FUNCTION "SINCRONIZZAZIONE ASSI" : VOID
TITLE =CICLO DI SINCRONIZZAZIONE ASSI
VERSION : 0.1

BEGIN
NETWORK
TITLE =INIZIO SINCRONIZZAZIONE
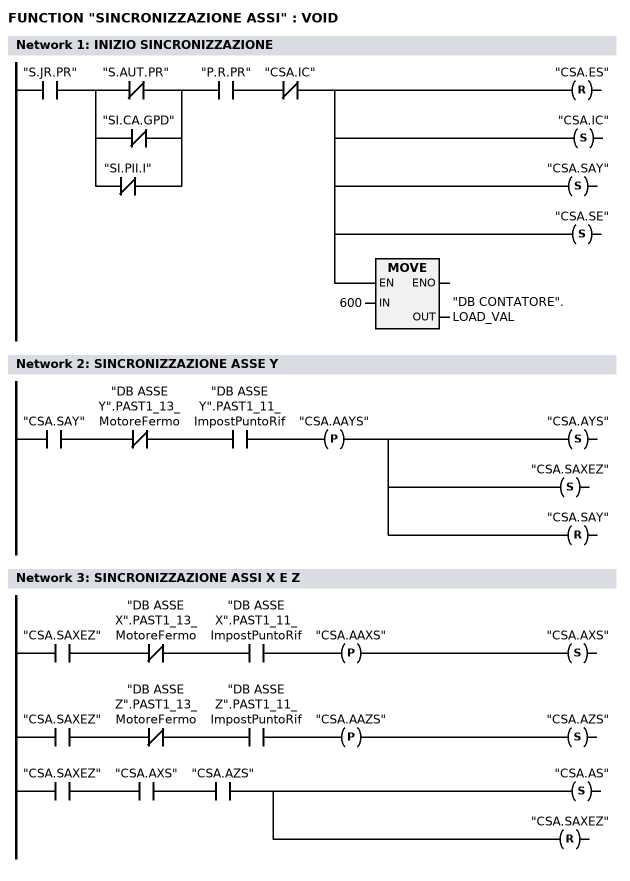
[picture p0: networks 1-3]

      U     "S.JR.PR";
      U(    ;
      ON    "S.AUT.PR";
      ON    "SI.CA.GPD";
      ON    "SI.PII.I";
      )     ;
      U     "P.R.PR";
      UN    "CSA.IC";
      R     "CSA.ES";
      S     "CSA.IC";
      S     "CSA.SAY";
      S     "CSA.SE";
      SPBN  ET01;
      L     600;
      T     "DB CONTATORE".LOAD_VAL;
ET01: NOP   0;

NETWORK
TITLE =SINCRONIZZAZIONE ASSE Y

      U     "CSA.SAY";
      UN    "DB ASSE Y".PAST1_13_MotoreFermo;
      U     "DB ASSE Y".PAST1_11_ImpostPuntoRif;
      FP    "CSA.AAYS";
      S     "CSA.AYS";
      S     "CSA.SAXEZ";
      R     "CSA.SAY";

NETWORK
TITLE =SINCRONIZZAZIONE ASSI X E Z

      U     "CSA.SAXEZ";
      UN    "DB ASSE X".PAST1_13_MotoreFermo;
      U     "DB ASSE X".PAST1_11_ImpostPuntoRif;
      FP    "CSA.AAXS";
      S     "CSA.AXS";
//---------------------------
      U     "CSA.SAXEZ";
      UN    "DB ASSE Z".PAST1_13_MotoreFermo;
      U     "DB ASSE Z".PAST1_11_ImpostPuntoRif;
      FP    "CSA.AAZS";
      S     "CSA.AZS";
//---------------------------
      U     "CSA.SAXEZ";
      U     "CSA.AXS";
      U     "CSA.AZS";
      S     "CSA.AS";
      R     "CSA.SAXEZ";

NETWORK
TITLE =SINCRONIZZAZIONE ENCODER

      U     "CSA.SE";
      U     "FP.SI.PCN";
      S     "L_DIRECT";
      S     "CSA.SOE";
      R     "CSA.SE";
//------------------------
      U     "CSA.SOE";
      UN    "L_DIRECT";
      SPBN  ET02;
      L     2047;
      T     "DB CONTATORE".LOAD_VAL;
      S     "L_PREPAR";
ET02: NOP   0;
//------------------------
      U     "CSA.SOE";
      UN    "L_DIRECT";
      U(    ;
      L     "DB CONTATORE".ACT_LOAD;
      L     1500;
      >=D   ;
      )     ;
      S     "CSA.ES";
      R     "CSA.SOE";

NETWORK
TITLE =CONCLUSIONE CICLO SINCRONIZZAZIONE
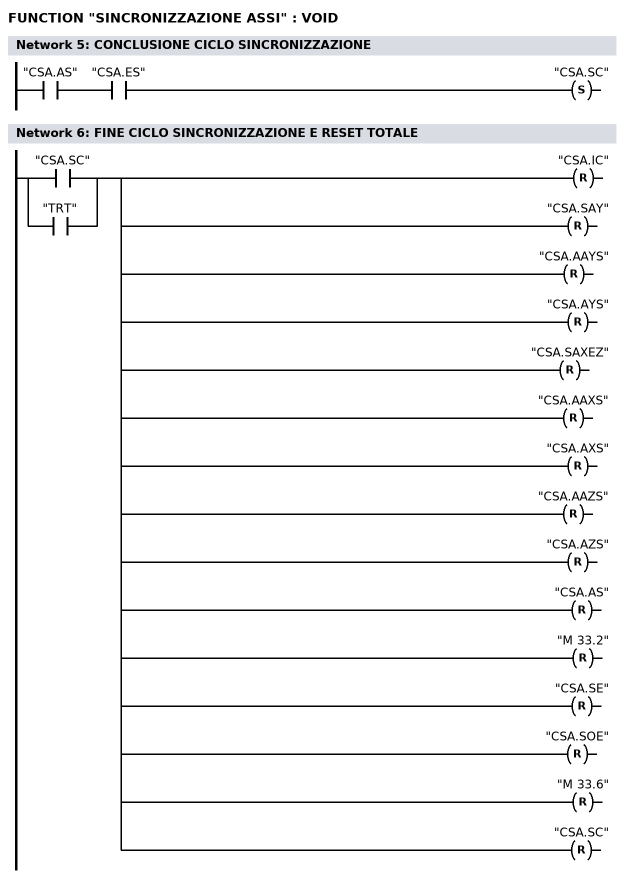
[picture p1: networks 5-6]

      U     "CSA.AS";
      U     "CSA.ES";
      S     "CSA.SC";

NETWORK
TITLE =FINE CICLO SINCRONIZZAZIONE E RESET TOTALE

      O     "CSA.SC";
      O     "TRT";
      R     "CSA.IC";
      R     "CSA.SAY";
      R     "CSA.AAYS";
      R     "CSA.AYS";
      R     "CSA.SAXEZ";
      R     "CSA.AAXS";
      R     "CSA.AXS";
      R     "CSA.AAZS";
      R     "CSA.AZS";
      R     "CSA.AS";
      R     "M      33.2";
      R     "CSA.SE";
      R     "CSA.SOE";
//      R     "CSA.ES"
      R     "M      33.6";
      R     "CSA.SC";



END_FUNCTION

